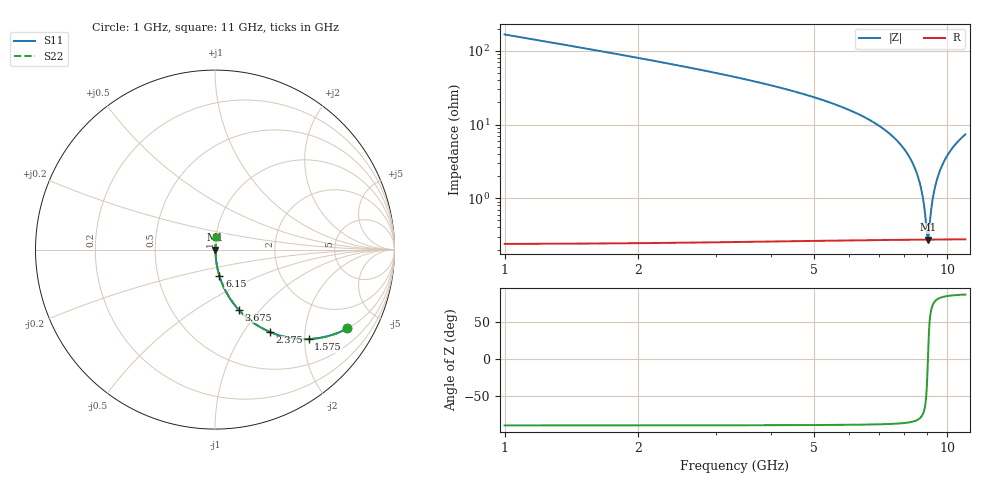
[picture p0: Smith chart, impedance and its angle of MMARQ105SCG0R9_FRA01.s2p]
! MMARQ105SCG0R9_FRA01  S-PARAMETER MODEL  ( General Type )
! Model Generated by TAIYO YUDEN Corporation (http://www.ty-top.com)
! Version 1.0
! TAIYO YUDEN Control No. 200326
! Copyright(c) 2020 TAIYO YUDEN CO.,LTD. All Rights Reserved.
! Product Description (link to TY-COMPAS)
! https://ds.yuden.co.jp/TYCOMPAS/or/detail?pn=MMARQ105SCG0R9BFRA01&u=M
! Products Name : Multilayer Ceramic Capacitors
! Characteristics :
!  Capacitance : 0.9 pF , Rated Voltage : 250V , TCC : CG / C0G
!  Case Size : 1.0 x 0.5 / 0.039 x 0.02 [mm/inch] , Thickness : 0.5 / 0.02 [mm/inch]
!  (Conditions: Temperature = 25 degC , DC Bias Current/Voltage = 0A / 0V)
! External Node Assignments :
!  1  o---| |---o  2
! GND o---------o GND
! Frequency Range : 1GHz  -  11GHz  [ 401 STEP ]
# MHz S RI R 50
! Freq[MHz].  S11 Real  S11 Imag  S21 Real  S21 Imag  S12 Real  S12 Imag  S22 Real  S22 Imag
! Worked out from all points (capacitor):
!   401 points, 1 GHz to 11 GHz, reference 50 ohm
!   read as one part in series: C = 937 fF near 1.05 GHz
!   lowest |Z| = 274 mohm at 9.05 GHz (marker M1)
!   series resonance near 9.05 GHz, so ESL is about 330 pH
!   S11 on the Smith chart (normalised r, x): 1 GHz: 1.00, -3.35; 1.575 GHz: 1.00, -2.09; 2.375 GHz: 1.00, -1.33; 3.675 GHz: 1.01, -0.77; 6.15 GHz: 1.01, -0.30; 11 GHz: 1.01, +0.15
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1000  0.7375 -0.4393  0.2625 0.4393  0.2625 0.4393  0.7375 -0.4393
1575  0.5222 -0.4984  0.4778 0.4984  0.4778 0.4984  0.5222 -0.4984
2375  0.3077 -0.4597  0.6923 0.4597  0.6923 0.4597  0.3077 -0.4597
2675  0.2521 -0.4321  0.7479 0.4321  0.7479 0.4321  0.2521 -0.4321
3675  0.1312 -0.3343  0.8688 0.3343  0.8688 0.3343  0.1312 -0.3343
4350  0.0846 -0.274  0.9154 0.274  0.9154 0.274  0.0846 -0.274
6000  0.027 -0.1538  0.973 0.1538  0.973 0.1538  0.027 -0.1538
6150  0.0241 -0.1446  0.9759 0.1446  0.9759 0.1446  0.0241 -0.1446
7675  0.00651 -0.0615  0.9935 0.0615  0.9935 0.0615  0.00651 -0.0615
8200  0.00408 -0.0368  0.9959 0.0368  0.9959 0.0368  0.00408 -0.0368
8575  0.00313 -0.0201  0.9969 0.0201  0.9969 0.0201  0.00313 -0.0201
8800  0.00284 -0.0105  0.9972 0.0105  0.9972 0.0105  0.00284 -0.0105
8900  0.00277 -0.00624  0.9972 0.00624  0.9972 0.00624  0.00277 -0.00624
9000  0.00273 -0.00207  0.9973 0.00207  0.9973 0.00207  0.00273 -0.00207
9050  0.00273 -3.39e-06  0.9973 3.39e-06  0.9973 3.39e-06  0.00273 -3.39e-06
9100  0.00274 0.00205  0.9973 -0.00205  0.9973 -0.00205  0.00274 0.00205
9225  0.00278 0.00714  0.9972 -0.00714  0.9972 -0.00714  0.00278 0.00714
9350  0.00288 0.0122  0.9971 -0.0122  0.9971 -0.0122  0.00288 0.0122
9600  0.00322 0.022  0.9968 -0.022  0.9968 -0.022  0.00322 0.022
9950  0.004 0.0354  0.996 -0.0354  0.996 -0.0354  0.004 0.0354
10425  0.00555 0.0528  0.9945 -0.0528  0.9945 -0.0528  0.00555 0.0528
11000  0.0081 0.0728  0.9919 -0.0728  0.9919 -0.0728  0.0081 0.0728
